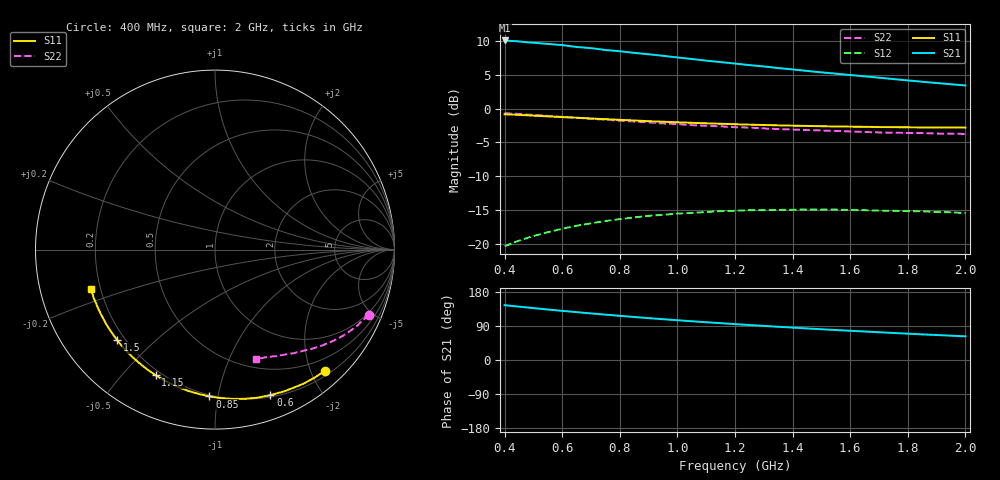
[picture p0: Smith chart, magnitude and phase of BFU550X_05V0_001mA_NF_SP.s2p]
! Filename:  P:\Prog\Test\Noise\ATS_data\Testdata_Net\BFU550X no attenuator noise\BFU550X_APG2013_44_C05_05p0V_001mA_NF_CM01_D.sf
! Date/Time: Fri 26/Jul/2013 14:37:11
! BFU550X_APG2013_44_C05_05p0V_1to10mA_NF_CM01_Bias1_R.sf
! Noise Parameter Data File
! BFU550X_APG2013_44_C05_05p0V_1to10mA_NF_CM01
! Date/time: Wed Jul 24 16:36:15 2013
! freq range =  0.4000 to  2.0000 GHz, 37 points
! bias range =  0.9950 to 10.0000 mA, 5 points
! bias supplies used: 1 1 0 0 0 0
! VAR bias_mode= 1  ! Specify V_out, I_out
! VAR bias_var = 1  ! Bias variable = I_out
! VAR V_out= 5.000000
! VAR I_out= 0.995000
! VAR V_in= 0.776600
! VAR I_in= 0.010701
! Device data file deembeded for feedlines and parallel
! Original file: \BFU550X no attenuator noise\BFU550X_APG2013_44_C05_05p0V_001mA_NF_CM01_R.sf
! Feed-files: PR005V01_100713_Feed1.s2p, PR005V01_100713_Feed2.s2p
! Parallel-file: PR005V01_100713_Par.s2p
# MHz S MA R 50
!  Freq-MHz  S11-mag  S11-arg  S21-mag  S21-arg  S12-mag  S12-arg  S22-mag  S22-arg
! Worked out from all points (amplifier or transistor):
!   37 points, 400 MHz to 2 GHz, reference 50 ohm
!   highest |S21| = 10.1 dB at 400 MHz (marker M1)
!   |S21| within 3 dB of that: start of sweep to 1.101 GHz
!   unconditionally stable (mu >= 1): nowhere
!   at 500 MHz: K = 0.13, MSG = 14.3 dB, |S12| = -18.9 dB
!   at 1.1 GHz: K = 0.27, MSG = 11.2 dB, |S12| = -15.3 dB
!   at 2 GHz: K = 0.49, MSG = 9.5 dB, |S12| = -15.5 dB
!   lowest NFmin = 0.59 dB at 460 MHz
!   S11 on the Smith chart (normalised r, x): 400 MHz: 0.28, -2.23; 600 MHz: 0.22, -1.43; 850 MHz: 0.19, -0.94; 1.15 GHz: 0.18, -0.62; 1.5 GHz: 0.17, -0.38; 2 GHz: 0.16, -0.15
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400  0.9109 -47.8  3.215 144.7  0.09559 60.0  0.93 -22.9
440  0.903 -52.3  3.176 141.6  0.1032 57.4  0.9185 -24.8
480  0.8949 -56.6  3.111 138.5  0.1101 54.9  0.9051 -26.7
500  0.8894 -58.8  3.093 136.9  0.1137 53.5  0.9018 -27.8
550  0.8787 -64.0  3.03 133.2  0.1213 50.5  0.8856 -30.0
600  0.8675 -69.2  2.971 129.7  0.1287 47.5  0.8713 -32.2
650  0.8585 -73.9  2.876 126.3  0.1355 44.8  0.858 -34.1
700  0.8473 -78.8  2.819 122.8  0.1413 42.0  0.8428 -36.2
750  0.8376 -83.3  2.732 119.7  0.1469 39.5  0.8299 -37.9
800  0.8279 -87.9  2.674 116.5  0.1518 37.0  0.816 -39.8
850  0.819 -92.2  2.601 113.5  0.1563 34.6  0.804 -41.4
900  0.8093 -96.4  2.539 110.5  0.1605 32.3  0.7933 -43.0
950  0.8017 -100.5  2.474 107.6  0.1633 30.0  0.7787 -44.8
1050  0.787 -108.1  2.342 102.2  0.1688 25.9  0.7569 -47.6
1150  0.7743 -115.3  2.221 97.2  0.1739 22.1  0.7415 -50.2
1200  0.768 -118.8  2.167 94.6  0.1748 20.2  0.7304 -51.7
1350  0.7536 -128.5  2.007 87.7  0.1777 15.1  0.7071 -55.4
1500  0.7424 -137.4  1.864 81.2  0.1787 10.5  0.69 -58.8
1600  0.7371 -143.0  1.781 77.1  0.1774 7.6  0.6782 -61.3
1750  0.7306 -150.7  1.661 71.3  0.1751 3.8  0.6651 -64.4
1850  0.7271 -155.5  1.588 67.6  0.1733 1.4  0.6603 -66.3
2000  0.7254 -162.4  1.49 62.5  0.1681 -1.8  0.65 -69.5
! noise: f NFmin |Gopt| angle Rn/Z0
400  0.6252  0.6154  28.72  0.3361
460  0.5891  0.6101  37.91  0.2867
600  0.6977  0.6406  46.83  0.3561
800  0.7664  0.6206  62.35  0.298
1000  0.8137  0.62  77.9  0.2674
1200  0.884  0.631  92.82  0.2226
1400  0.9306  0.6795  104.9  0.2268
1600  0.8765  0.6252  122  0.1072
1800  0.8566  0.5907  136.5  0.0912
2000  1.244  0.6465  147.5  0.078
